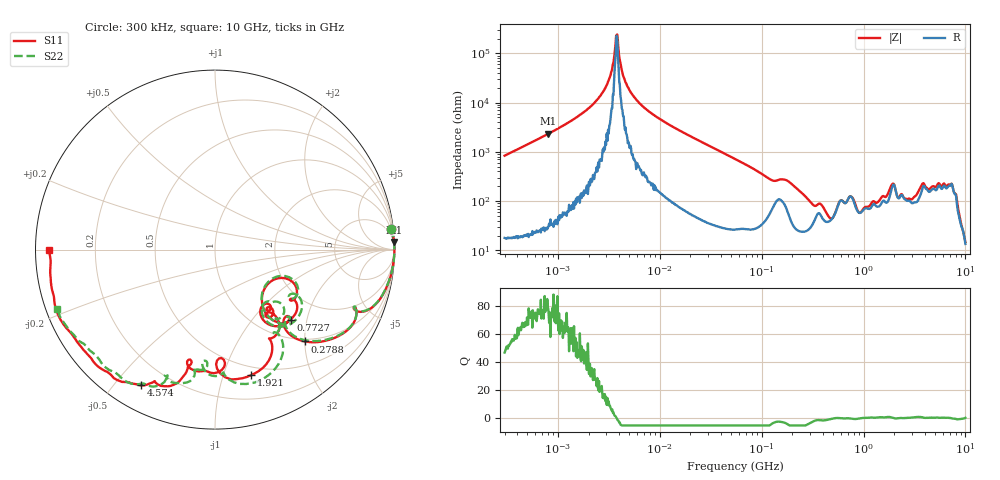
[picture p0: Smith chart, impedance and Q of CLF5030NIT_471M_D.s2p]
! S-Parameter Data Generated by TDK Corporation
! Copyright(C) 2019 TDK Corporation.
! All Rights Reserved.
! TDK P/N: CLF5030NIT-471M-D (Inductor)
! Property: L=470uH at 100kHz
! Size(LxWxT): 5.3x5x2.7mm
! Model Type: s2p (Touchstone File Format Version 1.0)
! Frequency: DC=Yes Start=0.3MHz Stop=10000MHz 802points Log-sweep
! Model Generated on May 10, 2019
! Port Assignments:
!  1 ---@@@--- 2
! Applicable Conditions:
!  Temperature = 25 degC
!  DC Bias Current = 0 A
!  Small Signal Operation
! Terms and conditions regarding TDK Simulation Models
! (1)This simulation model is being provided solely for informational purposes. Please refer to the specifications of the products in terms of detailed characteristics of such products.
! (2)In no event shall TDK Corporation of any of its subsidiaries be liable for any loss or damage arising, directly or indirectly,
!  From any information contained in this simulation model, including, but not limited to loss or damages arising from any inaccuracies, omissions or errors in connection with such information.
! (3)Any and all copyrights on this simulation model are owned by TDK Corporation.
!  Duplication or redistribution of this simulation model without prior written permission from TDK Corporation is prohibited.
! (4)This simulation model is subject to any modification or change without any prior notice.
! (5)Neither TDK Corporation nor any of its subsidiaries shall make any warranty, express or implied,
!  Including but not limited to the correctness, implied warranties of merchantability and fitness for a particular purpose with respect to this simulation models.
! (6)The use of this simulation model shall be deemed to have consented to the terms and conditions hereof.
# Hz S MA R 50
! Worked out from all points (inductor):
!   801 points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, 300 kHz to 10 GHz, reference 50 ohm
!   read as one part in series: L = 441 uH near 318.3 kHz
!   highest Q = 78 at 808.6 kHz (marker M1), where L = 460 uH
!   self-resonance near 3.777 MHz
!   S11 on the Smith chart (normalised r, x): 300 kHz: 1, +17; 278.8 MHz: 0.95, -2.00; 772.7 MHz: 1.38, -1.60; 1.921 GHz: 0.42, -1.24; 4.574 GHz: 0.10, -0.59; 10 GHz: 0.04, -0.00
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300000  0.9896 6.8  0.1182 -82.0  0.1182 -82.0  0.9894 6.8
808588  0.9982 2.4  0.04274 -86.8  0.04254 -86.8  0.9981 2.4
1713600  0.9993 0.9  0.0168 -88.0  0.01685 -87.6  0.9993 0.9
2972263  0.9996 0.2  0.004665 -86.1  0.004711 -84.7  0.9996 0.1
3777497  0.9995 -0.1  0.0004263 -14.9  0.0003502 -13.6  0.9996 -0.2
4363314  0.9995 -0.3  0.002817 81.0  0.002766 81.5  0.9996 -0.3
5044683  0.9995 -0.5  0.005589 85.6  0.005594 84.8  0.9995 -0.5
9671944  0.9991 -1.6  0.0206 86.5  0.02059 86.5  0.9991 -1.6
5.477226e7  0.9856 -10.1  0.1369 77.8  0.1369 77.8  0.9852 -10.1
1.855783e8  0.8737 -27.5  0.344 51.3  0.3439 51.3  0.873 -27.2
2.787792e8  0.7153 -45.7  0.5688 33.1  0.5687 33.1  0.716 -45.0
3.126428e8  0.6112 -48.7  0.6144 22.6  0.6144 22.6  0.6147 -47.9
5.344909e8  0.3861 -24.4  0.6121 -20.4  0.6122 -20.4  0.3805 -23.1
7.726947e8  0.5743 -42.8  0.4268 -16.7  0.4268 -16.7  0.5971 -40.2
9.216398e8  0.4197 -52.9  0.5948 -26.3  0.5949 -26.3  0.42 -51.6
1.767019e9  0.6531 -60.9  0.3571 -88.2  0.3569 -88.3  0.6513 -54.4
1.920785e9  0.7282 -74.1  0.2329 -84.8  0.2327 -84.9  0.7599 -66.8
2.924554e9  0.6311 -103.5  0.2876 -98.1  0.2869 -98.1  0.6757 -97.0
3.816223e9  0.8116 -110.3  0.1229 -125.0  0.1229 -124.8  0.7774 -108.0
4.574322e9  0.8606 -118.5  0.1341 -127.5  0.1343 -127.6  0.7892 -110.9
7.763894e9  0.9465 -157.5  0.03268 -127.4  0.03286 -127.9  0.9236 -150.0
1e10  0.924 -179.8  0.04686 -91.7  0.0466 -91.8  0.9378 -159.4
